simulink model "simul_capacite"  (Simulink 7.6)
settings: Solver=ode15s  StartTime=0.0  StopTime=2  RelTol=1e-3
InitFcn:
  | clear all, clc
  | R1=0.1e3;
  | R2=0.001*R1;
  | R=R1;
  | C=1e-3;
StopFcn:
  | close all, clc
  | load simul_capacite.mat
  | plot(x(1,:),x(2,:),x(1,:),x(3,:))
  | title('Capacité simulée et son circuit équivalent')
  | axis([0 2 -0.2 1.2])
  | xlabel('temps')
  | grid
  | delete *.mat
undefined symbols (not defined in the file or in its folder): sigbuilder_block
libraries: fl_lib x12, nesl_utility x4, elec_lib x2

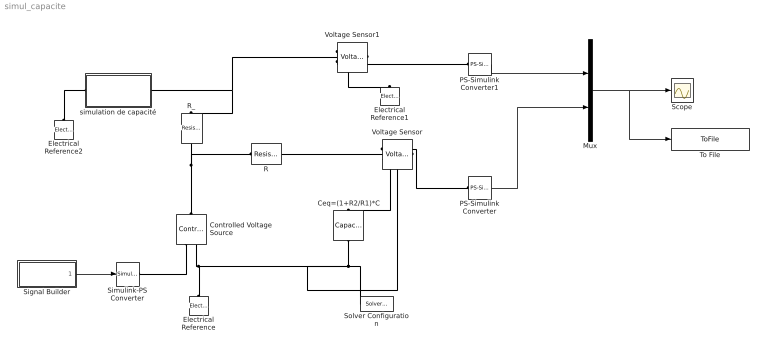
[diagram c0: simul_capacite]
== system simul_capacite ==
  Ceq=(1+R2/R1)*C : fl_lib/Electrical/Electrical Elements/Capacitor  DialogController=NetworkEngine.DynNeDlgSource  SystemSampleTime=-1  c=(1+R2/R1)*C F  v0=0 V  r=1e-22 Ohm  g=0 1/Ohm  i_Log=off  v_Log=off  vc_Log=off  LocalVarNames=|i|v|vc  LocalVarDescs=|i|v|Internal variable for voltage across capacitor term  LocalVarLogging=[0 0 0]
  Controlled Voltage Source : fl_lib/Electrical/Electrical Sources/Controlled Voltage Source  DialogController=NetworkEngine.DynNeDlgSource  SystemSampleTime=-1  i_Log=off  v_Log=off  LocalVarNames=|i|v  LocalVarDescs=|i|v  LocalVarLogging=[0 0]
  Electrical Reference : fl_lib/Electrical/Electrical Elements/Electrical Reference  DialogController=NetworkEngine.DynNeDlgSource  SystemSampleTime=-1  i_Log=off  LocalVarNames=|i  LocalVarDescs=|i  LocalVarLogging=[]
  Electrical Reference1 : fl_lib/Electrical/Electrical Elements/Electrical Reference  DialogController=NetworkEngine.DynNeDlgSource  SystemSampleTime=-1  i_Log=off  LocalVarNames=|i  LocalVarDescs=|i  LocalVarLogging=[]
  Electrical Reference2 : fl_lib/Electrical/Electrical Elements/Electrical Reference  DialogController=NetworkEngine.DynNeDlgSource  SystemSampleTime=-1  i_Log=off  LocalVarNames=|i  LocalVarDescs=|i  LocalVarLogging=[]
  Mux : Mux  Inputs=2
  PS-Simulink Converter : nesl_utility/PS-Simulink Converter  DialogController=NetworkEngine.DynNeUtilDlgSource  SystemSampleTime=-1  PhysicalDomain=network_engine_domain  LeftPortType=input  RightPortType=output  SubClassName=ps_output  Unit=1  AffineConversion=off
  PS-Simulink Converter1 : nesl_utility/PS-Simulink Converter  DialogController=NetworkEngine.DynNeUtilDlgSource  SystemSampleTime=-1  PhysicalDomain=network_engine_domain  LeftPortType=input  RightPortType=output  SubClassName=ps_output  Unit=1  AffineConversion=off
  R : fl_lib/Electrical/Electrical Elements/Resistor  DialogController=NetworkEngine.DynNeDlgSource  SystemSampleTime=-1  R=R Ohm  i_Log=off  v_Log=off  LocalVarNames=|i|v  LocalVarDescs=|i|v  LocalVarLogging=[0 0]
  R_ : fl_lib/Electrical/Electrical Elements/Resistor  DialogController=NetworkEngine.DynNeDlgSource  SystemSampleTime=-1  R=R Ohm  i_Log=off  v_Log=off  LocalVarNames=|i|v  LocalVarDescs=|i|v  LocalVarLogging=[0 0]
  Scope : Scope
  Signal Builder : Subsystem  Tag=STV Subsys  LoadFcn=sigbuilder_block('load',[195.75 6.75 550.5 399.75 ]);  StartFcn=sigbuilder_block('start');  StopFcn=sigbuilder_block('stop');  ClipboardFcn=sigbuilder_block('clipboard');
  Simulink-PS Converter : nesl_utility/Simulink-PS Converter  DialogController=NetworkEngine.DynNeUtilDlgSource  SystemSampleTime=-1  PhysicalDomain=network_engine_domain  LeftPortType=input  RightPortType=output  SubClassName=ps_input  Unit=1  AffineConversion=off  InputFilterTimeConstant=.001  UdotUserProvided=0
  Solver Configuration : nesl_utility/Solver Configuration  DialogController=NetworkEngine.DynNeUtilDlgSource  SystemSampleTime=-1  PhysicalDomain=network_engine_domain  LeftPortType=input  RightPortType=generic  SubClassName=solver  Accelerate=off  Profile=off  ResidualTolerance=1e-9  MaxNonlinIter=12  MaxModeIter=2  DoFixedCost=off  UseLocalSampling=off  DoDC=off  LinearAlgebra=Sparse  LocalSolverSampleTime=.001  LocalSolverChoice=NE_BACKWARD_EULER_ADVANCER  UseLocalSolver=off
  To File : ToFile  Filename=simul_capacite  MatrixName=x
  Voltage Sensor : fl_lib/Electrical/Electrical Sensors/Voltage Sensor  DialogController=NetworkEngine.DynNeDlgSource  SystemSampleTime=-1  i1_Log=off  v1_Log=off  LocalVarNames=|i1|v1  LocalVarDescs=|i1|v1  LocalVarLogging=[0 0]
  Voltage Sensor1 : fl_lib/Electrical/Electrical Sensors/Voltage Sensor  DialogController=NetworkEngine.DynNeDlgSource  SystemSampleTime=-1  i1_Log=off  v1_Log=off  LocalVarNames=|i1|v1  LocalVarDescs=|i1|v1  LocalVarLogging=[0 0]
  simulation de capacité : Subsystem
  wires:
  PS-Simulink Converter1/1 -> Mux/1
  PS-Simulink Converter/1 -> Mux/2
  Mux/1 -> Scope/1, To File/1
  Signal Builder/1(Signal 1) -> Simulink-PS Converter/1
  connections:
  Controlled Voltage Source/RConn1 -- Simulink-PS Converter/RConn1
  Ceq=(1+R2/R1)*C/RConn1 -- Voltage Sensor/RConn2 -- Electrical Reference/LConn1 -- Controlled Voltage Source/RConn2 -- Solver Configuration/RConn1
  Voltage Sensor1/LConn1 -- R_/LConn1 -- simulation de capacité/LConn1
  Voltage Sensor/RConn1 -- PS-Simulink Converter/LConn1
  Voltage Sensor1/RConn1 -- PS-Simulink Converter1/LConn1
  Voltage Sensor1/RConn2 -- Electrical Reference1/LConn1
  Voltage Sensor/LConn1 -- Ceq=(1+R2/R1)*C/LConn1 -- R/RConn1
  Controlled Voltage Source/LConn1 -- R/LConn1 -- R_/RConn1
  Electrical Reference2/LConn1 -- simulation de capacité/RConn1

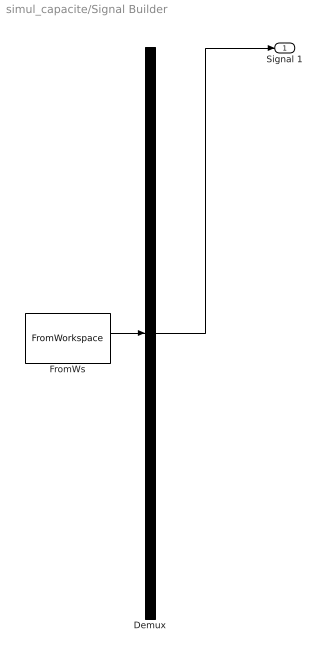
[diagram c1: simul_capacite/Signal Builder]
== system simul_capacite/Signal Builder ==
  Demux : Demux  Tag=STV Demux  Outputs=1
  FromWs : FromWorkspace  Tag=STV FromWs  VariableName=tuvar  SampleTime=0  SigBuilderData=DataTag0  VnvData=DataTag1
  Signal 1 : Outport  Tag=STV Outport
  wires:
  Demux/1 -> Signal 1/1
  FromWs/1 -> Demux/1

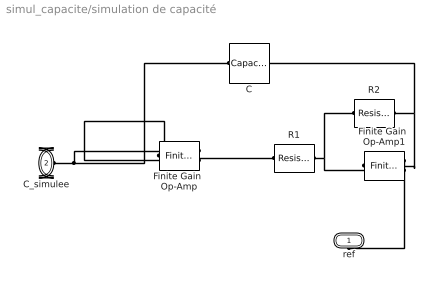
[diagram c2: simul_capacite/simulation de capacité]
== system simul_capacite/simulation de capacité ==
  C : fl_lib/Electrical/Electrical Elements/Capacitor  DialogController=NetworkEngine.DynNeDlgSource  SystemSampleTime=-1  c=C F  v0=0 V  r=1e-22 Ohm  g=0 1/Ohm  i_Log=off  v_Log=off  vc_Log=off  LocalVarNames=|i|v|vc  LocalVarDescs=|i|v|Internal variable for voltage across capacitor term  LocalVarLogging=[0 0 0]
  Finite Gain  Op-Amp : elec_lib/Integrated Circuits/Finite Gain Op-Amp  DialogController=NetworkEngine.DynNeDlgSource  SystemSampleTime=-1  A=1000  Rin=1e+6 Ohm  Rout=100 Ohm  Vmin=-15 V  Vmax=15 V  LocalVarLogging=[]
  Finite Gain  Op-Amp1 : elec_lib/Integrated Circuits/Finite Gain Op-Amp  DialogController=NetworkEngine.DynNeDlgSource  SystemSampleTime=-1  A=1000  Rin=1e+6 Ohm  Rout=100 Ohm  Vmin=-15 V  Vmax=15 V  LocalVarLogging=[]
  R1 : fl_lib/Electrical/Electrical Elements/Resistor  DialogController=NetworkEngine.DynNeDlgSource  SystemSampleTime=-1  R=R1 Ohm  i_Log=off  v_Log=off  LocalVarNames=|i|v  LocalVarDescs=|i|v  LocalVarLogging=[0 0]
  R2 : fl_lib/Electrical/Electrical Elements/Resistor  DialogController=NetworkEngine.DynNeDlgSource  SystemSampleTime=-1  R=R2 Ohm  i_Log=off  v_Log=off  LocalVarNames=|i|v  LocalVarDescs=|i|v  LocalVarLogging=[0 0]
  ref : PMIOPort  Port=1  Side=Right
  C_simulee : PMIOPort  Port=2  Side=Left
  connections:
  Finite Gain  Op-Amp/RConn1 -- R1/LConn1 -- Finite Gain  Op-Amp/LConn2
  R1/RConn1 -- Finite Gain  Op-Amp1/LConn2 -- R2/LConn1
  C_simulee/RConn1 -- Finite Gain  Op-Amp/LConn1 -- C/RConn1
  R2/RConn1 -- Finite Gain  Op-Amp1/RConn1 -- C/LConn1
  Finite Gain  Op-Amp1/LConn1 -- ref/RConn1
